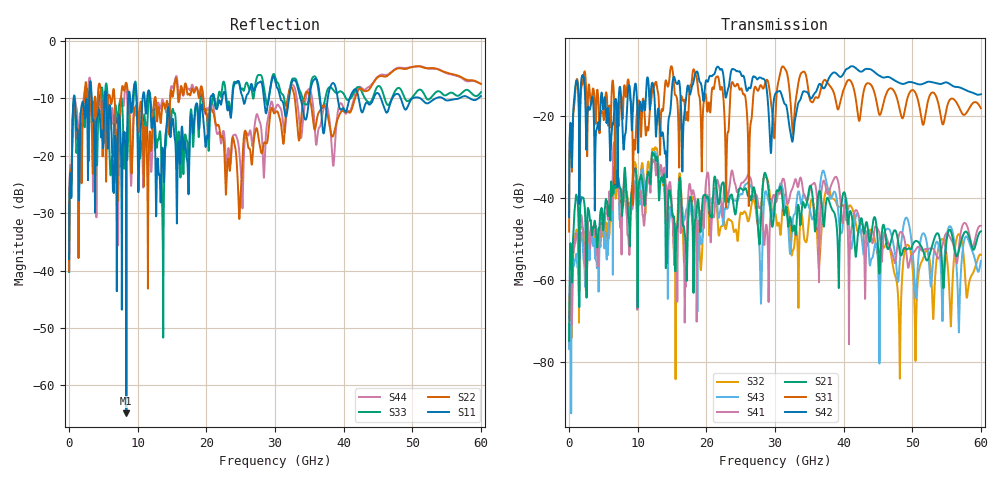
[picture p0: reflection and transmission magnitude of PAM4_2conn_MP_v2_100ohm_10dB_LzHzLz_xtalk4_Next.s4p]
! Info: Touchstone file created by Circ.  Input file=FAB50GbE_2conn_Midplane_Examax_Topo2_v2_100ohm_10dB_LzHzLz.circ
# Hz S RI R 50
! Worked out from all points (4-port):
!   6000 points, 10 MHz to 60 GHz, reference 50 ohm
!   strongest paths, dB at 10 MHz, 15.01 GHz, 30.01 GHz, 45.01 GHz, 60 GHz:
!     S42: -44.7, -13.0, -14.7, -9.9, -14.7
!     S31: -48.2, -8.2, -22.9, -18.5, -18.1
!     S21: -74.9, -43.4, -41.5, -51.9, -48.1
!     S41: -67.8, -42.9, -39.8, -47.7, -46.8
!     S43: -70.8, -43.6, -40.1, -55.7, -55.3
!     S32: -74.3, -44.6, -43.7, -54.0, -53.8
!   lowest |S11| = -64.9 dB at 8.35 GHz (marker M1), VSWR 1.00, Z = 49.9 - j0.0055 ohm
!   |S11| at or under -10 dB: 5.431 GHz to 8.635 GHz (3.203 GHz wide, 45.5 % of centre); 11.81 GHz to 20.61 GHz (8.8 GHz wide, 54.3 % of centre); 54.44 GHz to 56.89 GHz (2.453 GHz wide, 4.41 % of centre)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
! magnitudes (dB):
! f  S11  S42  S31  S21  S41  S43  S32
! 10 MHz  -38.0  -44.7  -48.2  -74.9  -67.8  -70.8  -74.3
! 1.03 GHz  -14.5  -11.6  -11.8  -39.3  -48.8  -53.8  -48.6
! 8.35 GHz  -64.9  -21.5  -14.6  -38.2  -40.6  -43.3  -38.5
! 24.85 GHz  -7.7  -9.1  -13.6  -37.6  -37.6  -39.2  -45.0
! 37.75 GHz  -9.6  -11.1  -12.1  -40.1  -39.0  -38.1  -37.6
! 48.14 GHz  -9.5  -11.9  -18.1  -52.7  -48.6  -56.5  -76.0
! 60 GHz  -9.6  -14.7  -18.1  -48.1  -46.8  -55.3  -53.8
